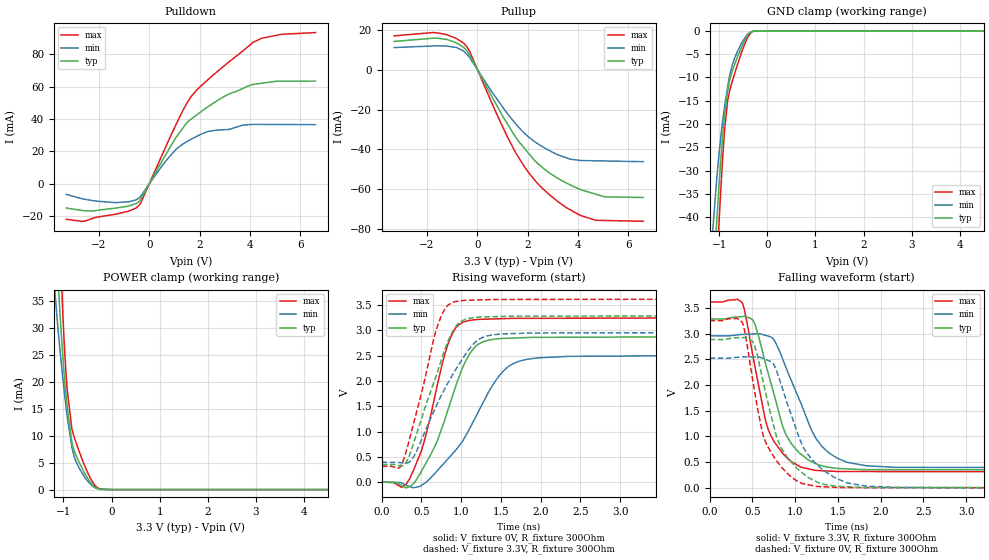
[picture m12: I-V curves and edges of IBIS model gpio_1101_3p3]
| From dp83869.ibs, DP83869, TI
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|   gpio_1101_3p3 Model
[Model]   gpio_1101_3p3
Model_type   I/O
Polarity   Non-Inverting
Enable   Active-Low
Vinl = 0.7
Vinh = 1.7
Vmeas = 1.65
Vref = 0
Cref = 2pF
Rref = 100000
|   typ   min   max
C_comp   1.10585pF   1.10585pF   1.45739pF
| Where Nom  PVT is Nominal Process, 3.3V,  27C
|   Fast PVT is Strong Process,  3.63V, -40C
|   Slow PVT is Weak Process,   2.97V, 125C
[Voltage Range]   3.3   2.97   3.63
|Junction Temperature
[Temperature Range]   27   125   -40
[Pullup Reference]   3.3   2.97   3.63
[Pulldown Reference]   0   -0   -0
[Power Clamp Reference]   3.3   2.97   3.63
[GND Clamp Reference]   0   0   0
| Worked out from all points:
|   slope of the pulldown table from 0 to 0.495 V, typ, clamps not added: 36.1 ohm
|   slope of the pullup table from 0 to 0.495 V, typ, clamps not added: 42.1 ohm
|   GND clamp passes 1 mA (typ) near -0.41 V on its own axis
|   POWER clamp passes 1 mA (typ) near -0.41 V on its own axis
|   falling waveform, V_fixture 3.3V, R_fixture 300Ohm: 20-80 % time 317ps typ, 400ps min, 264ps max; typ from 3.29 V to 0.35 V
|   rising waveform, V_fixture 0V, R_fixture 300Ohm: 20-80 % time 403ps typ, 578ps min, 303ps max; typ from 0 V to 2.88 V
|   rising waveform, V_fixture 3.3V, R_fixture 300Ohm: 20-80 % time 377ps typ, 501ps min, 306ps max; typ from 0.35 V to 3.29 V
|   falling waveform, V_fixture 0V, R_fixture 300Ohm: 20-80 % time 323ps typ, 387ps min, 277ps max; typ from 2.89 V to 0 V
[Pulldown]
|   Voltage   I(typ)   I(min)   I(max)
-3.3V     -15.05mA   -6.588mA   -22.04mA
-2.543V   -16.74mA   -9.704mA   -23.09mA
-1.345V   -15.12mA   -11.7mA    -18.91mA
-510.8mV  -12.13mA   -9.848mA   -14.82mA
-332.6mV  -9.344mA   -7.451mA   -11.59mA
1.079V    29mA       21.5mA     37.16mA
1.47V     37.34mA    25.78mA    49.21mA
1.922V    43mA       29.61mA    58.51mA
2.885V    53.15mA    33.3mA     71.73mA
4.128V    61.4mA     36.68mA    87.48mA
5.241V    63.38mA    36.6mA     92.35mA
6.6V      63.44mA    36.5mA     93.45mA
[GND Clamp]
|   Voltage   I(typ)   I(min)   I(max)
-3.3V     -489.2mA   -422.2mA   -556.8mA
-1.128V   -53.94mA   -41.75mA   -66.49mA
-1.053V   -40.94mA   -31.89mA   -50.85mA
-1.004V   -32.91mA   -26.23mA   -40.88mA
-914.8mV  -20.88mA   -18.15mA   -24.96mA
-886mV    -17.91mA   -16.01mA   -20.9mA
-824.7mV  -12.98mA   -11.96mA   -14.96mA
-737.5mV  -8.884mA   -7.637mA   -11.14mA
-632.6mV  -5.898mA   -4.664mA   -7.616mA
-450.4mV  -1.653mA   -1.242mA   -2.33mA
-341.5mV  -279.4uA   -241.7uA   -417.8uA
6.6V      0A         0A         0A
[Pullup]
|   Voltage   I(typ)   I(min)   I(max)
-3.3V     14.34mA    11.25mA    17.14mA
-1.661V   15.94mA    12.09mA    18.72mA
-570.2mV  11.63mA    9.688mA    13.74mA
-306.9mV  7.711mA    6.276mA    9.45mA
741mV     -17.06mA   -13.87mA   -21.25mA
1.47V     -32.73mA   -26.26mA   -40.35mA
1.917V    -40.07mA   -32.35mA   -49.5mA
2.55V     -48.65mA   -38.29mA   -59.11mA
3.164V    -54.26mA   -42.5mA    -65.87mA
4.127V    -60.31mA   -45.59mA   -73.33mA
5.058V    -63.84mA   -45.81mA   -75.74mA
6.6V      -64.2mA    -46.16mA   -76.16mA
[POWER Clamp]
|   Voltage   I(typ)   I(min)   I(max)
-3.3V     592.7mA    473.7mA    711.1mA
-1.183V   53.33mA    37.6mA     74.54mA
-1.164V   49.45mA    35.35mA    69.48mA
-1.121V   40.99mA    30.62mA    58.01mA
-1.071V   32.56mA    25.84mA    45.66mA
-1.013V   24.62mA    20.7mA     32.69mA
-952.4mV  18.17mA    15.83mA    22.43mA
-922.7mV  15.44mA    13.63mA    18.69mA
-824.7mV  8.834mA    7.855mA    11.3mA
-668.2mV  4.976mA    3.912mA    6.986mA
-331.6mV  381.5uA    308.5uA    658.7uA
6.6V      0A         0A         0A
[Ramp]
R_load = 300
|   typ   min   max
dV/dt_r   1.72601/4.01632e-10   1.50543/5.77069e-10   1.94854/3.02171e-10
dV/dt_f   1.76231/3.1393e-10   1.53885/3.98878e-10   1.98179/2.63959e-10
[Falling Waveform]
V_fixture = 3.3V
V_fixture_min = 2.97V
V_fixture_max = 3.63V
R_fixture = 300Ohm
C_fixture = 0F
|   Time   V(typ)   V(min)   V(max)
0s        3.287V     2.957V     3.616V
380.4ps   3.331V     2.983V     3.597V
507.7ps   3.258V     2.992V     2.548V
644.8ps   2.471V     2.97V      1.38V
699.8ps   2.136V     2.943V     1.073V
884.9ps   1.063V     2.372V     616.9mV
1.06ns    665mV      1.673V     409.2mV
1.316ns   428.3mV    802.4mV    333.3mV
1.615ns   368.8mV    494.2mV    317.7mV
5ns       349.5mV    392.6mV    312.8mV
[Rising Waveform]
V_fixture = 0V
V_fixture_min = 0V
V_fixture_max = 0V
R_fixture = 300Ohm
C_fixture = 0F
|   Time   V(typ)   V(min)   V(max)
0s        173.6uV    264.3uV    176.9uV
248.1ps   -67.35mV   -16.95mV   -103.6mV
349.1ps   -86.03mV   -88.03mV   60.89mV
531.9ps   305.7mV    -32.14mV   789.1mV
827.4ps   1.399V     449.9mV    2.698V
1.025ns   2.286V     829.8mV    3.162V
1.216ns   2.727V     1.391V     3.215V
1.475ns   2.834V     2.094V     3.227V
1.733ns   2.851V     2.391V     3.235V
5ns       2.877V     2.509V     3.248V
[Rising Waveform]
V_fixture = 3.3V
V_fixture_min = 2.97V
V_fixture_max = 3.63V
R_fixture = 300Ohm
C_fixture = 0F
|   Time   V(typ)   V(min)   V(max)
0s        349.5mV    392.6mV    312.8mV
260.8ps   319.8mV    379.9mV    388.7mV
403.5ps   783.8mV    505.7mV    1.176V
691.3ps   2.126V     1.519V     3.037V
792.5ps   2.615V     1.842V     3.417V
884.4ps   2.952V     2.103V     3.547V
989.2ps   3.167V     2.369V     3.582V
1.176ns   3.253V     2.765V     3.598V
1.397ns   3.268V     2.91V      3.607V
5ns       3.286V     2.957V     3.616V
[Falling Waveform]
|Gnd
V_fixture = 0V
V_fixture_min = 0V
V_fixture_max = 0V
R_fixture = 300Ohm
C_fixture = 0F
|   Time   V(typ)   V(min)   V(max)
0s        2.886V     2.523V     3.254V
378.5ps   2.922V     2.546V     3.227V
505.3ps   2.838V     2.545V     2.073V
612.6ps   2.162V     2.525V     1.11V
678.8ps   1.677V     2.48V      805.5mV
820.9ps   828.4mV    2.086V     444.5mV
1.07ns    311.3mV    880.3mV    93.07mV
1.336ns   70.88mV    333.7mV    21.3mV
1.828ns   6.112mV    34.95mV    4.912mV
5ns       167.6uV    249.6uV    174uV
